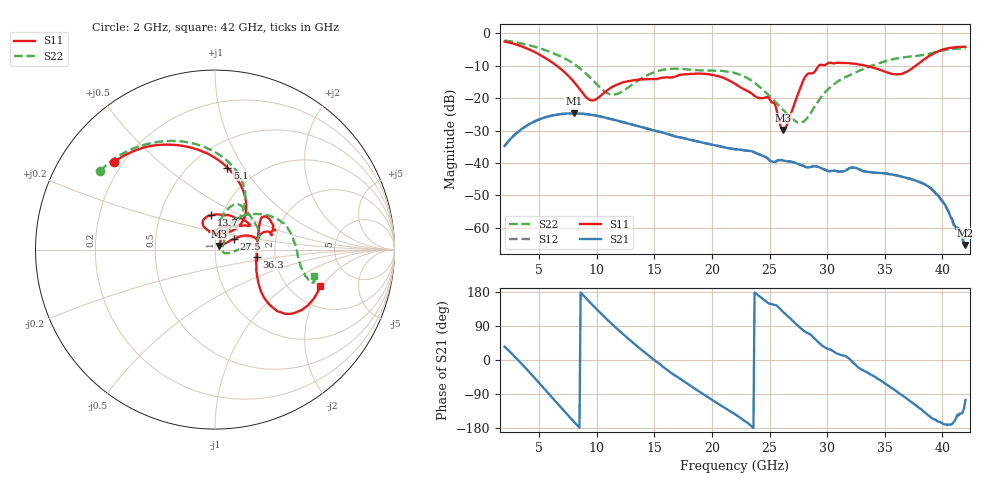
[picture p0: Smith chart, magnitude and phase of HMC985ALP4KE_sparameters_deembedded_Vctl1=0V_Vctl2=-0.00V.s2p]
!s2p File: Measurements: S11, S21, S12, S22
# GHz S dB R 50.0
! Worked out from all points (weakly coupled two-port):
!   401 points, 2 GHz to 42 GHz, reference 50 ohm
!   highest |S21| = -24.69 dB at 8 GHz (marker M1); lowest = -65.3 dB at 42 GHz (marker M2)
!   lowest |S11| = -29.8 dB at 26.2 GHz (marker M3), VSWR 1.07, Z = 52.5 + j2.2 ohm
!   |S11| at or under -10 dB: 6.525 GHz to 29.28 GHz (22.75 GHz wide, 127 % of centre); 33.34 GHz to 37.69 GHz (4.35 GHz wide, 12.2 % of centre)
!   |S22| runs from -27.6 to -2.2 dB; largest |S21 - S12| = 0.00013
!   S11 on the Smith chart (normalised r, x): 2 GHz: 0.16, +0.36; 5.1 GHz: 0.73, +0.85; 13.7 GHz: 0.89, +0.35; 27.5 GHz: 1.22, +0.15; 36.3 GHz: 1.59, -0.14; 42 GHz: 2.90, -1.91
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2  -2.54 139.3  -34.74 35.2  -34.73 35.3  -2.20 145.7
3.5  -4.06 111.3  -29.49 -10.7  -29.49 -10.7  -3.15 122.0
5.1  -6.71 81.3  -26.41 -64.1  -26.42 -64.2  -4.68 97.7
8  -14.91 44.7  -24.69 -162.3  -24.70 -162.4  -9.39 60.1
8.7  -18.09 51.5  -24.80 174.8  -24.80 174.7  -11.28 54.6
9.7  -20.70 87.4  -25.23 143.0  -25.23 143.0  -14.63 51.8
11.3  -16.64 115.9  -26.49 95.3  -26.50 95.3  -18.86 67.9
13.7  -14.29 96.7  -28.73 31.6  -28.74 31.5  -14.31 77.2
15.4  -13.94 73.0  -30.32 -9.3  -30.32 -9.3  -11.53 68.4
19.4  -12.51 34.7  -33.87 -93.3  -33.88 -93.3  -11.47 34.2
22  -15.56 52.2  -35.71 -143.1  -35.74 -143.2  -12.25 13.0
25  -20.24 97.5  -39.20 148.4  -39.21 148.3  -19.38 -5.1
26.2  -29.84 40.6  -39.26 126.3  -39.23 126.2  -23.72 -18.4
27.5  -18.43 29.5  -40.32 89.2  -40.28 89.2  -27.46 -5.4
28.1  -13.37 20.6  -41.11 74.3  -41.16 74.3  -26.80 20.4
28.7  -12.32 12.7  -41.06 63.1  -41.10 63.2  -23.83 40.3
31  -9.10 23.3  -42.65 15.3  -42.61 15.3  -14.67 57.6
35.4  -12.27 12.4  -43.40 -69.8  -43.45 -69.7  -8.30 26.3
36.3  -12.58 -10.1  -44.07 -89.3  -44.05 -88.8  -7.62 18.3
39.1  -6.53 -44.9  -48.08 -153.9  -48.23 -152.9  -6.09 -12.5
40.2  -4.84 -37.5  -52.62 -170.2  -52.77 -167.3  -5.15 -18.1
42  -4.14 -19.1  -65.26 -105.6  -65.25 -101.3  -4.87 -14.9
